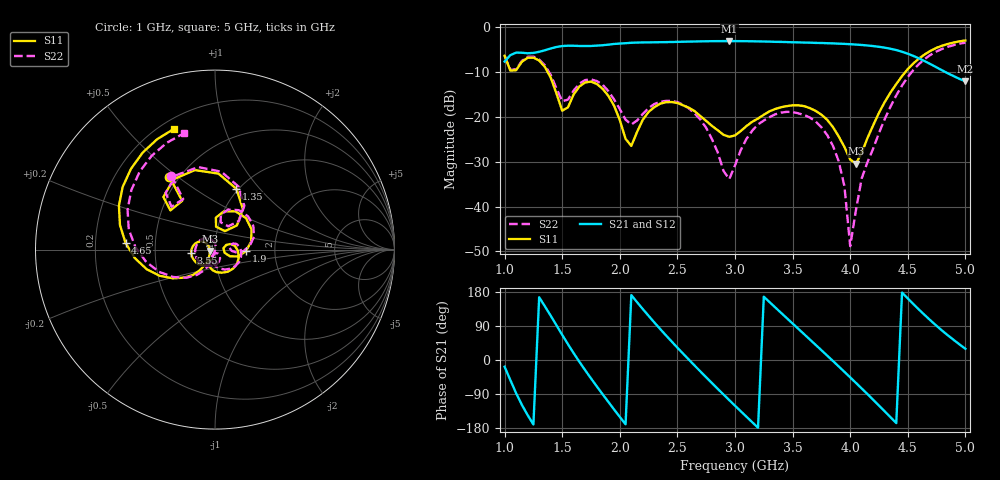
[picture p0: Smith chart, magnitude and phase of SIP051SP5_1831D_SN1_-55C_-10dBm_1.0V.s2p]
# GHz  S  dB  R  50
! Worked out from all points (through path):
!   81 points, 1 GHz to 5 GHz, reference 50 ohm
!   highest |S21| = -3.11 dB at 2.95 GHz (marker M1); lowest = -12.1 dB at 5 GHz (marker M2)
!   lowest |S11| = -30.4 dB at 4.05 GHz (marker M3), VSWR 1.06, Z = 47.2 - j0.724 ohm
!   |S11| at or under -10 dB: 1.374 GHz to 4.479 GHz (3.106 GHz wide, 106 % of centre)
!   |S22| runs from -48.8 to -3.5 dB; largest |S21 - S12| = 0.0018
!   S11 on the Smith chart (normalised r, x): 1 GHz: 0.44, +0.47; 1.35 GHz: 0.98, +0.76; 1.9 GHz: 1.41, -0.03; 3.55 GHz: 0.76, -0.03; 4.65 GHz: 0.33, +0.03; 5 GHz: 0.25, +0.68
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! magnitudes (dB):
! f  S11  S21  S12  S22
! 1 GHz  -6.4  -7.7  -7.7  -6.4
! 1.05 GHz  -9.7  -6.2  -6.2  -9.6
! 1.35 GHz  -8.9  -5.2  -5.2  -8.5
! 1.5 GHz  -18.6  -4.2  -4.2  -16.5
! 1.7 GHz  -12.3  -4.2  -4.2  -11.8
! 1.9 GHz  -15.3  -3.9  -3.9  -14.2
! 2.1 GHz  -26.5  -3.5  -3.5  -21.7
! 2.35 GHz  -17.1  -3.4  -3.4  -16.6
! 2.7 GHz  -19.9  -3.2  -3.2  -20.6
! 2.95 GHz  -24.4  -3.1  -3.1  -33.9
! 3 GHz  -24.2  -3.1  -3.1  -30.8
! 3.2 GHz  -20.4  -3.2  -3.2  -21.7
! 3.55 GHz  -17.4  -3.4  -3.4  -19.2
! 3.7 GHz  -18.7  -3.5  -3.5  -21.0
! 3.9 GHz  -24.4  -3.7  -3.7  -29.9
! 3.95 GHz  -26.7  -3.7  -3.7  -35.5
! 4 GHz  -29.5  -3.8  -3.8  -48.8
! 4.05 GHz  -30.4  -3.9  -3.9  -40.8
! 4.1 GHz  -28.0  -4.0  -4.0  -33.7
! 4.35 GHz  -14.6  -4.8  -4.8  -17.7
! 4.65 GHz  -6.0  -7.6  -7.6  -7.1
! 5 GHz  -3.0  -12.1  -12.1  -3.5
